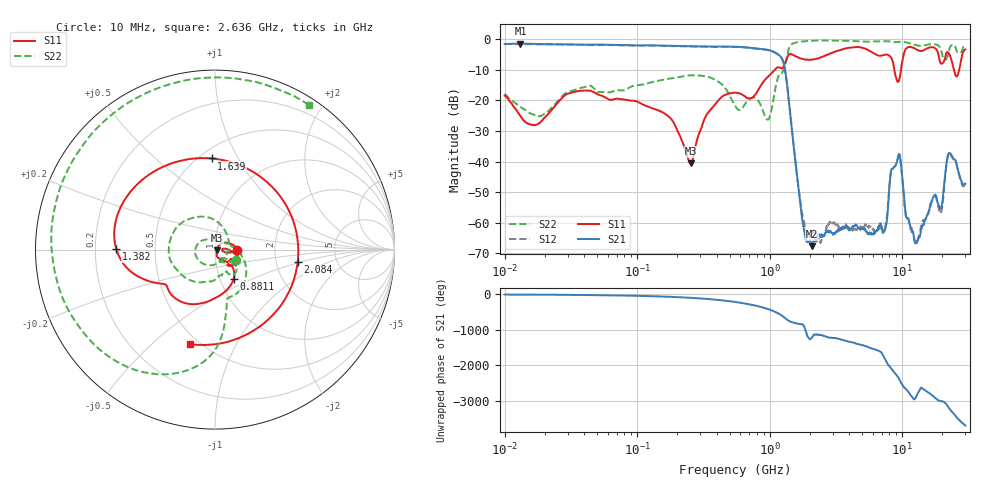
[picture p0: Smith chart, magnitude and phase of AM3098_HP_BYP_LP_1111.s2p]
!Agilent Technologies,E8364B,MY43040894,A.07.50.67
!Agilent E8364B: A.07.50.67
!Date: Wednesday, June 17, 2020 09:22:03
!Correction: S11(Full 2 Port(1,2))
!S21(Full 2 Port(1,2))
!S12(Full 2 Port(1,2))
!S22(Full 2 Port(1,2))
!S2P File: Measurements: S11, S21, S12, S22:Log Frequency Sweep
# Hz S  dB  R 50
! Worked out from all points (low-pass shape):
!   1601 points, 10 MHz to 30 GHz, reference 50 ohm
!   highest |S21| = -1.39 dB at 13.17 MHz (marker M1); lowest = -67.7 dB at 2.073 GHz (marker M2)
!   |S21| within 3 dB of the highest: start of sweep to 1.113 GHz
!   lowest |S11| = -40.6 dB at 253.4 MHz (marker M3), VSWR 1.02, Z = 50.9 - j0.311 ohm
!   |S11| at or under -10 dB: start of sweep to 1.09 GHz; 8.725 GHz to 9.785 GHz (1.06 GHz wide, 11.5 % of centre); 24.63 GHz to 26.91 GHz (2.281 GHz wide, 8.85 % of centre)
!   |S22| runs from -26.3 to -0.3 dB; largest |S21 - S12| = 0.014
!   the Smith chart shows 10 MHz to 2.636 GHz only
!   S11 on the Smith chart (normalised r, x): 10 MHz: 1.27, -0.01; 881.1 MHz: 1.16, -0.39; 1.382 GHz: 0.29, +0.00; 1.639 GHz: 0.57, +0.78; 2.084 GHz: 2.64, -0.48; 2.636 GHz: 0.45, -0.67
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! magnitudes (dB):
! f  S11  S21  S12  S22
! 10 MHz  -18.4  -1.5  -1.5  -17.8
! 13.17 MHz  -25.1  -1.4  -1.5  -22.1
! 38.04 MHz  -16.8  -1.7  -1.7  -15.8
! 144.7 MHz  -23.2  -2.0  -2.0  -13.5
! 253.4 MHz  -40.6  -2.2  -2.3  -11.8
! 337.1 MHz  -24.4  -2.3  -2.4  -12.2
! 547.7 MHz  -17.5  -2.4  -2.5  -21.7
! 881.1 MHz  -14.3  -3.2  -3.3  -22.9
! 1.226 GHz  -9.5  -5.9  -6.0  -11.1
! 1.382 GHz  -5.2  -18.3  -18.4  -3.6
! 1.639 GHz  -5.9  -47.4  -47.5  -0.9
! 2.073 GHz  -6.6  -67.7  -64.2  -0.4
! 2.084 GHz  -6.6  -67.0  -63.3  -0.4
! 2.636 GHz  -5.3  -63.5  -63.0  -0.4
! 7.207 GHz  -5.1  -63.3  -62.8  -0.6
! 7.926 GHz  -5.2  -51.4  -50.5  -0.6
! 9.49 GHz  -13.3  -37.5  -37.8  -0.8
! 12.81 GHz  -3.3  -66.8  -66.6  -1.9
! 19.7 GHz  -7.9  -55.2  -56.7  -3.7
! 22.67 GHz  -4.8  -37.2  -37.3  -3.3
! 25.82 GHz  -12.1  -41.0  -41.3  -4.0
! 30 GHz  -3.3  -47.3  -47.9  -2.1
